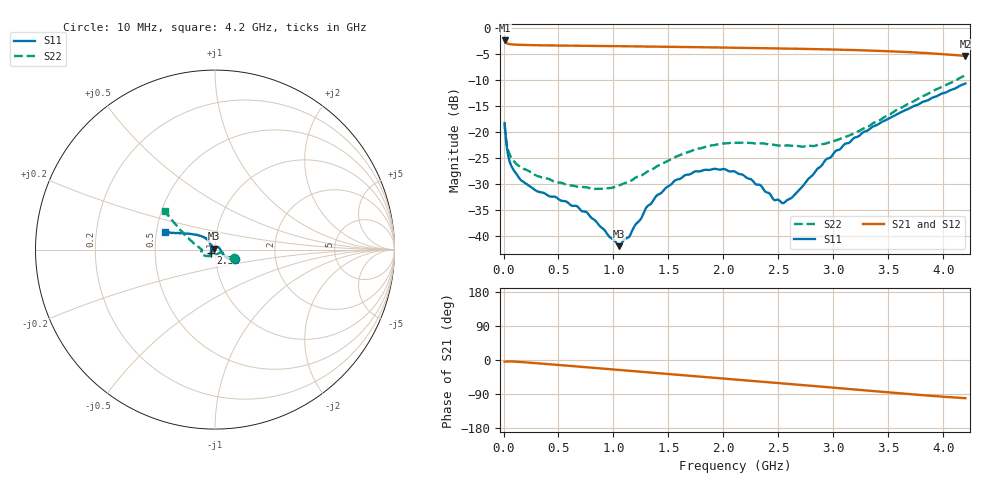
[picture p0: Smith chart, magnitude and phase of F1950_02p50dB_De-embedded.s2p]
! Integrated Device Technology
! Corporate Headquarters
! 6024 Silver Creek Valley Road
! San Jose, CA 95138  USA
! Phone:  1-408-284-8200
! Toll Free:  1-800-223-1366
! Webpage:  http://www.idt.com/
! Timing and RF Division
! 515 Groton Road, Suite 102
! Westford, MA 01886-6024
! Device:  F1950
! Description: 7-bit 0.25 dB Digital Step Attenuator
! Frequency:  150.0 -  4000.00 MHz
! Package:  4x4 mm Thin QFN Plastic Package: 24 pin
! Ports:  2 RF, 12 DC
!  Pin  1  = D0
!  Pin  2  = VDD
!  Pin  3  = Vmode
!  Pin  4  = GND
!  Pin  5  = RF1  =  Port 1
!  Pin  6  = GND
!  Pin  7  = GND
!  Pin  8  = GND
!  Pin  9  = GND
!  Pin 10  = GND
!  Pin 11  = GND
!  Pin 12  = GND
!  Pin 13  = GND
!  Pin 14  = RF2  =  Port 2
!  Pin 15  = GND
!  Pin 16  = LE
!  Pin 17  = CLK
!  Pin 18  = DATE
!  Pin 19  = D6
!  Pin 20  = D5
!  Pin 21  = D4
!  Pin 22  = D3
!  Pin 23  = D2
!  Pin 24  = D1
! State:  10
! Atten State:  2.50 dB
! Voltage:  +5.00 Volts
! Current:  Not Measured mA
! Data:  The device was measured on a the F195X evaluation board which has
!  individual transmission lines to the RF pins.  Data was collected
!  using a calibrated network analyzer.  The evaluation board was
!  de-embedded using a TRL calibration technique.
!  The reference plane is the edge of the package pin.
! Misc:  Board 2019
!  Action Tracker AT0250
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# GHz S dB R 50
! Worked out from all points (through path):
!   420 points, 10 MHz to 4.2 GHz, reference 50 ohm
!   highest |S21| = -2.38 dB at 10 MHz (marker M1); lowest = -5.4 dB at 4.2 GHz (marker M2)
!   group delay of S21, straight-line fit = 66.5 ps
!   lowest |S11| = -42.0 dB at 1.05 GHz (marker M3), VSWR 1.02, Z = 49.4 + j0.533 ohm
!   |S11| at or under -10 dB: start of sweep to end of sweep
!   |S22| runs from -31.0 to -9.1 dB; largest |S21 - S12| = 0.00083
!   S11 on the Smith chart (normalised r, x): 10 MHz: 1.24, -0.13; 2.32 GHz: 0.95, -0.04; 4.2 GHz: 0.56, +0.12
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0.01  -18.29 -25.2  -2.38 -4.3  -2.38 -4.3  -18.62 -23.7
0.06  -25.97 -29.3  -3.11 -3.7  -3.11 -3.7  -24.51 -26.7
0.16  -29.31 -12.8  -3.23 -5.3  -3.23 -5.3  -26.83 -22.9
0.3  -31.36 8.2  -3.30 -8.4  -3.30 -8.5  -28.42 -24.6
0.47  -32.50 30.4  -3.35 -12.4  -3.35 -12.4  -29.68 -28.9
0.71  -35.24 58.8  -3.41 -18.1  -3.41 -18.1  -30.62 -44.4
0.91  -38.72 90.0  -3.45 -22.8  -3.45 -22.8  -30.96 -67.0
1.05  -42.00 137.2  -3.49 -26.1  -3.49 -26.2  -30.30 -88.4
1.14  -40.26 174.4  -3.51 -28.3  -3.51 -28.3  -29.57 -100.9
1.3  -34.52 -152.9  -3.55 -32.1  -3.54 -32.1  -27.75 -120.2
1.41  -32.02 -143.6  -3.58 -34.7  -3.58 -34.7  -26.45 -130.4
1.56  -29.35 -137.3  -3.62 -38.3  -3.62 -38.3  -24.85 -141.2
1.74  -27.62 -132.4  -3.67 -42.6  -3.67 -42.6  -23.38 -151.0
1.92  -27.10 -130.4  -3.73 -46.9  -3.72 -47.0  -22.52 -158.5
2.11  -27.71 -131.2  -3.79 -51.5  -3.79 -51.5  -22.10 -164.1
2.32  -30.16 -142.5  -3.86 -56.5  -3.86 -56.5  -22.21 -168.7
2.46  -33.10 -162.0  -3.91 -59.8  -3.90 -59.8  -22.49 -171.2
2.55  -33.66 176.3  -3.93 -62.0  -3.93 -62.0  -22.63 -174.0
2.81  -28.35 130.5  -4.04 -68.3  -4.04 -68.4  -22.72 -179.5
3.1  -22.39 128.3  -4.18 -75.5  -4.18 -75.6  -21.05 173.1
3.51  -17.34 142.1  -4.46 -85.6  -4.46 -85.6  -16.68 159.1
4.2  -10.67 160.6  -5.37 -100.8  -5.37 -100.8  -9.11 142.7
